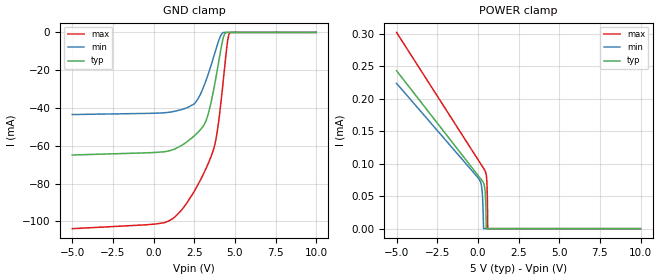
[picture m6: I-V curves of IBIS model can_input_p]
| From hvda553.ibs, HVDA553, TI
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|   can_input Model
[Model]   can_input_p
Model_type   Input
Vinl = 0.4
Vinh = 1.15
|   typ   min   max
|   (nom PVT)   (fast PVT)   (slow PVT)
 C_comp   8.003e-12   7.913e-12   8.671e-12
| Where nom  PVT is Nominal Process, 5V, 27C
|   Fast PVT is Strong Process,  5.33V, -40C
|   Slow PVT is Weak Process,   4.68V, 150C
[Voltage Range]   5   4.68   5.33
|Junction Temperature
[Temperature Range]   27   150   -40
[Power Clamp Reference]   5   4.68   5.33
[GND Clamp Reference]   0   0   0
[GND Clamp]
|   Voltage   I(typ)   I(min)   I(max)
-5V       -64.89mA   -43.48mA   -103.9mA
100mV     -63.53mA   -42.77mA   -101.4mA
1.284V    -61.74mA   -41.78mA   -97.79mA
2.46V     -55.02mA   -38.03mA   -84.61mA
3.068V    -49.37mA   -28.89mA   -74.77mA
3.37V     -42.71mA   -21.67mA   -69.07mA
3.695V    -30.06mA   -12.75mA   -61.54mA
3.99V     -15.9mA    -4.607mA   -47.48mA
4.295V    -2.371mA   -66.21uA   -24.18mA
4.557V    0A         0A         -3.831mA
4.663V    0A         0A         -385.2uA
9.995V    0A         0A         0A
[POWER Clamp]
|   Voltage   I(typ)   I(min)   I(max)
-5V       242.9uA    223.5uA    301.8uA
100mV     79uA       75.09uA    102.6uA
269.7mV   73.44uA    55.28uA    95.94uA
353.9mV   69.87uA    0A         92.63uA
447.3mV   56.96uA    0A         88.62uA
485mV     37.35uA    0A         86.19uA
515mV     1.551uA    0A         82.73uA
553.9mV   0A         0A         71.49uA
580.5mV   0A         0A         50.9uA
607.2mV   0A         0A         2.785uA
617.8mV   0A         0A         0A
9.995V    0A         0A         0A
